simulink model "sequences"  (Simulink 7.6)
settings: Solver=ode15s  StartTime=0.0  StopTime=2/60  FixedStep=Ts  RelTol=1e-3
InitFcn:
  | clc
  | a=exp(j*2*pi/3);
  | Ts=5e-5;
undefined symbols (not defined in the file or in its folder): Angle, Magnitude
libraries: powerlib x4, powerlib_extras x1

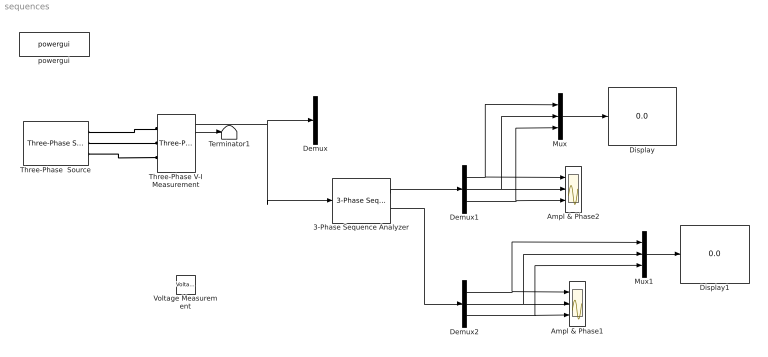
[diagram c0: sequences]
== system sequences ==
  3-Phase Sequence Analyzer : powerlib_extras/Measurements/3-Phase Sequence Analyzer  DialogController=POWERSYS.PowerSysDialog  SystemSampleTime=-1  f1=60  n=1  seq=Positive Negative Zero
  Ampl & Phase1 : Scope  NumInputPorts=3
  Ampl & Phase2 : Scope  NumInputPorts=3
  Demux : Demux  Outputs=3
  Demux1 : Demux  Outputs=3
  Demux2 : Demux  Outputs=3
  Display : Display
  Display1 : Display
  Mux : Mux  Inputs=3
  Mux1 : Mux  Inputs=3
  Terminator1 : Terminator
  Three-Phase V-I Measurement : powerlib/Measurements/Three-Phase V-I Measurement  DialogController=POWERSYS.PowerSysDialog  SystemSampleTime=-1  VoltageMeasurement=phase-to-ground  SetLabelV=off  LabelV=Vabc  Vpu=off  VpuLL=off  CurrentMeasurement=yes  SetLabelI=off  LabelI=Iabc  Ipu=off  Pbase=100e6  Vbase=500e3  OutputType=Magnitude-Angle  PhasorSimulation=off  PSBequivalent=0
  Three-Phase  Source : powerlib/Electrical Sources/Three-Phase Source  DialogController=POWERSYS.PowerSysDialog  SystemSampleTime=-1  Voltage=220*sqrt(3)/sqrt(2)  PhaseAngle=0  Frequency=60  InternalConnection=Yg  SpecifyImpedance=off  Resistance=0.8929  Inductance=1e-6  ShortCircuitLevel=100e6  BaseVoltage=25e3  XRratio=1e-12
  Voltage Measurement : powerlib/Measurements/Voltage Measurement  DialogController=POWERSYS.PowerSysDialog  SystemSampleTime=-1  PhasorSimulation=off  OutputType=Complex  PSBequivalent=0
  powergui : powerlib/powergui  Priority=1  SystemSampleTime=-1  SimulationMode=Continuous  SampleTime=Ts  frequency=60  SPID=off  DisableSnubberDevices=off  DisableRonSwitches=off  DisableVfSwitches=off  SwTol=0  Interpol=off  frequencyindice=60  echomessages=off  HookPort=off  DisplayEquations=off  FunctionMessages=off  EnableUseOfTLC=off  x0status=blocks  RestoreLinks=warning  ResistiveCurrentMeasurement=off  Ylog=off  Xlog=on  ShowGrid=off  save=off  variable=ZData  ZoomFFT=off  StartTime=0.0  cycles=1  DisplayStyle=1  FreqAxis=off  MaxFrequency=1000  frequencyindicesteady=1  display=off  methode=off
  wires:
  Three-Phase V-I Measurement/2 -> Terminator1/1
  Three-Phase V-I Measurement/1 -> Demux/1, 3-Phase Sequence Analyzer/1
  3-Phase Sequence Analyzer/1 -> Demux1/1
  Demux1/1 -> Ampl & Phase2/1, Mux/1
  Demux1/2 -> Ampl & Phase2/2, Mux/2
  Demux1/3 -> Ampl & Phase2/3, Mux/3
  Mux/1 -> Display/1
  3-Phase Sequence Analyzer/2 -> Demux2/1
  Demux2/1 -> Ampl & Phase1/1, Mux1/1
  Demux2/2 -> Ampl & Phase1/2, Mux1/2
  Demux2/3 -> Ampl & Phase1/3, Mux1/3
  Mux1/1 -> Display1/1
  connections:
  Three-Phase  Source/RConn1 -- Three-Phase V-I Measurement/LConn1
  Three-Phase  Source/RConn2 -- Three-Phase V-I Measurement/LConn2
  Three-Phase  Source/RConn3 -- Three-Phase V-I Measurement/LConn3
